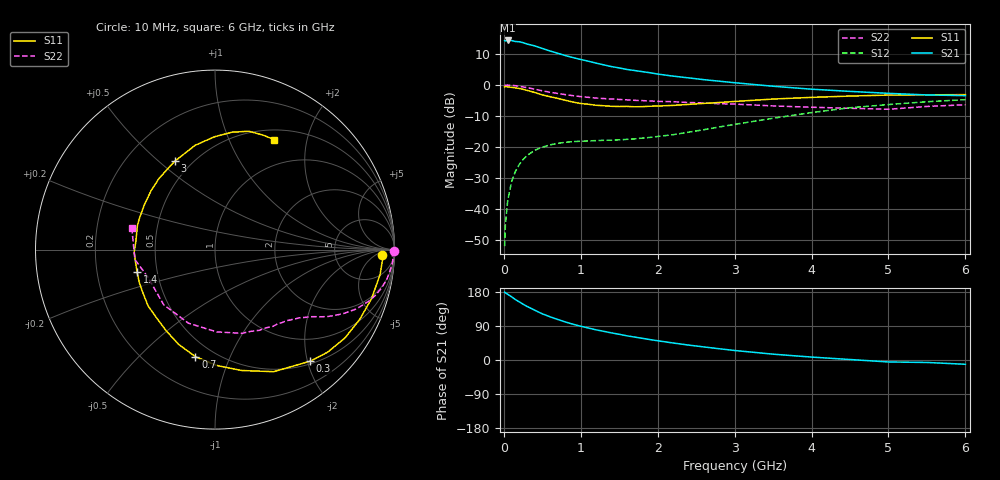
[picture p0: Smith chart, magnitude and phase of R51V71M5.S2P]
! SIEMENS Small Signal Semiconductors
! BFR183
! Si NPN RF Bipolar Junction Transistor in SOT23
! VCE = 1.75 V  IC = 1.5 mA
! Common Emitter S-Parameters:  May  1996
# GHz  S  MA  R  50
!  f  S11  S21  S12  S22
! GHz  MAG  ANG  MAG  ANG  MAG  ANG  MAG  ANG
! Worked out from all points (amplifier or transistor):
!   36 points, 10 MHz to 6 GHz, reference 50 ohm
!   highest |S21| = 14.3 dB at 50 MHz (marker M1)
!   |S21| within 3 dB of that: start of sweep to 551.9 MHz
!   unconditionally stable (mu >= 1): 1.481 GHz to 2.934 GHz
!   at 250 MHz: K = 0.19, MSG = 18.9 dB, |S12| = -24.1 dB
!   at 1.4 GHz: K = 0.96, MSG = 11.9 dB, |S12| = -17.8 dB
!   at 6 GHz: K = 0.94, MSG = 0.6 dB, |S12| = -4.8 dB
!   S11 on the Smith chart (normalised r, x): 10 MHz: 24, -10; 300 MHz: 0.55, -2.05; 700 MHz: 0.40, -0.75; 1.4 GHz: 0.38, -0.12; 3 GHz: 0.41, +0.56; 6 GHz: 0.62, +1.49
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0.01  0.9309 -1.7  5.191 179.0  0.0025 94.4  0.9971 -0.6
0.02  0.9352 -3.3  5.127 177.2  0.0055 90.2  0.9878 -1.4
0.05  0.9304 -8.5  5.215 173.4  0.0135 84.2  0.9935 -3.5
0.1  0.914 -17.4  5.198 166.9  0.0272 80.4  0.9822 -6.9
0.15  0.895 -25.8  5.02 159.6  0.04 75.3  0.9706 -10.1
0.2  0.8758 -34.1  4.97 153.4  0.0518 70.3  0.9506 -13.2
0.25  0.8494 -42.2  4.807 147.3  0.0624 66.0  0.9273 -16.1
0.3  0.8173 -49.5  4.572 141.5  0.0723 62.4  0.9042 -18.5
0.4  0.7548 -64.3  4.267 131.6  0.0881 55.6  0.8551 -22.7
0.5  0.6897 -77.6  3.875 121.8  0.0989 50.0  0.8033 -26.2
0.6  0.6452 -89.3  3.53 114.1  0.1078 45.6  0.7619 -28.8
0.7  0.6064 -100.4  3.242 107.0  0.1139 42.2  0.7285 -30.8
0.9  0.5278 -121.0  2.76 94.3  0.1217 38.0  0.6701 -33.9
1.1  0.4872 -139.9  2.409 84.3  0.1248 36.5  0.6298 -36.8
1.4  0.4518 -164.0  1.974 71.5  0.1284 36.9  0.5924 -40.6
1.8  0.4461 167.9  1.637 57.2  0.1387 42.3  0.558 -45.8
2.2  0.467 147.1  1.386 44.9  0.1573 48.1  0.536 -52.9
3  0.5407 114.6  1.085 25.1  0.2307 53.1  0.4901 -72.2
3.5  0.5915 100.8  0.951 15.4  0.2897 50.3  0.4583 -88.9
4.5  0.661 81.7  0.786 1.3  0.4282 37.7  0.4197 -133.0
5.5  0.6917 67.3  0.689 -6.5  0.5355 22.3  0.4495 -172.9
6  0.6962 61.7  0.671 -11.3  0.5784 12.8  0.4782 165.7
